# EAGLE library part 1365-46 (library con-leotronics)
DUAL ROW STRAIGHT HEADER 1364 SERIES. 1.27mm x 1.27mm. Without Fixing Post. SMT Source: http://www.leotronics.co.uk/Conexcon/Data%20Sheets/sec.%20A/1364ing.pdf
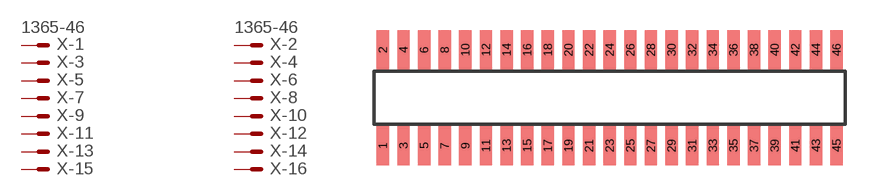
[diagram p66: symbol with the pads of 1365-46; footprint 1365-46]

Designator prefix X; gates -1=MVAL -2=MVAL -3=M -4=M -5=M -6=M -7=M -8=M -9=M -10=M -11=M -12=M -13=M -14=M -15=M -16=M -17=M -18=M -19=M -20=M -21=M -22=M -23=M -24=M -25=M -26=M -27=M -28=M -29=M -30=M -31=M -32=M -33=M -34=M -35=M -36=M -37=M -38=M -39=M -40=M -41=M -42=M -43=M -44=M -45=M -46=M

## 1365-46 (OC_FARNELL: unknown; OC_NEWARK: unknown)  [1365-46]
1  -1:S  pas
2  -2:S  pas
3  -3:S  pas
4  -4:S  pas
5  -5:S  pas
6  -6:S  pas
7  -7:S  pas
8  -8:S  pas
9  -9:S  pas
10  -10:S  pas
11  -11:S  pas
12  -12:S  pas
13  -13:S  pas
14  -14:S  pas
15  -15:S  pas
16  -16:S  pas
17  -17:S  pas
18  -18:S  pas
19  -19:S  pas
20  -20:S  pas
21  -21:S  pas
22  -22:S  pas
23  -23:S  pas
24  -24:S  pas
25  -25:S  pas
26  -26:S  pas
27  -27:S  pas
28  -28:S  pas
29  -29:S  pas
30  -30:S  pas
31  -31:S  pas
32  -32:S  pas
33  -33:S  pas
34  -34:S  pas
35  -35:S  pas
36  -36:S  pas
37  -37:S  pas
38  -38:S  pas
39  -39:S  pas
40  -40:S  pas
41  -41:S  pas
42  -42:S  pas
43  -43:S  pas
44  -44:S  pas
45  -45:S  pas
46  -46:S  pas

## Footprint 1365-46 (pad centres in mm)
DUAL ROW STRAIGHT HEADER 1364 SERIES. 1.27mm x 1.27mm. Without Fixing Post. SMT Source: http://www.leotronics.co.uk/Conexcon/Data%20Sheets/sec.%20A/1364ing.pdf
smd 0.76 x 2.4: 1 -13.97,-2.95; 2 -13.97,2.95; 3 -12.7,-2.95; 4 -12.7,2.95; 5 -11.43,-2.95; 6 -11.43,2.95; 7 -10.16,-2.95; 8 -10.16,2.95; 9 -8.89,-2.95; 10 -8.89,2.95; 11 -7.62,-2.95; 12 -7.62,2.95; 13 -6.35,-2.95; 14 -6.35,2.95; 15 -5.08,-2.95; 16 -5.08,2.95; 17 -3.81,-2.95; 18 -3.81,2.95; 19 -2.54,-2.95; 20 -2.54,2.95; 21 -1.27,-2.95; 22 -1.27,2.95; 23 0,-2.95; 24 0,2.95; 25 1.27,-2.95; 26 1.27,2.95; 27 2.54,-2.95; 28 2.54,2.95; 29 3.81,-2.95; 30 3.81,2.95; 31 5.08,-2.95; 32 5.08,2.95; 33 6.35,-2.95; 34 6.35,2.95; 35 7.62,-2.95; 36 7.62,2.95; 37 8.89,-2.95; 38 8.89,2.95; 39 10.16,-2.95; 40 10.16,2.95; 41 11.43,-2.95; 42 11.43,2.95; 43 12.7,-2.95; 44 12.7,2.95; 45 13.97,-2.95; 46 13.97,2.95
